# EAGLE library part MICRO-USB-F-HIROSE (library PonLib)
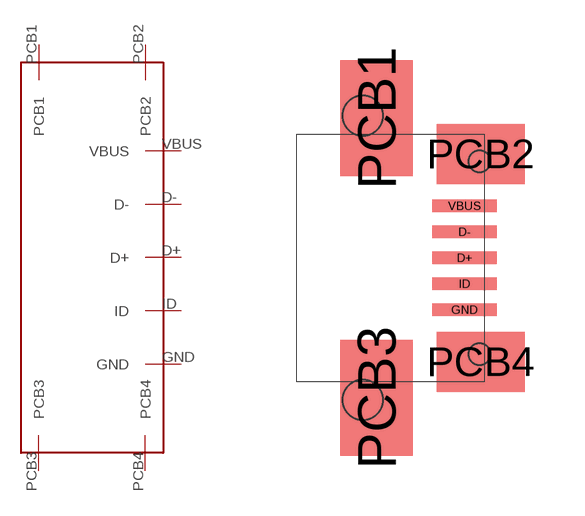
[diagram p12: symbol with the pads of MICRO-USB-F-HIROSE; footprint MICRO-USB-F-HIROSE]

Designator prefix -

## MICRO-USB-F-HIROSE  [MICRO-USB-F-HIROSE]
D+  D+
D-  D-
GND  GND
ID  ID
PCB1  PCB1
PCB2  PCB2
PCB3  PCB3
PCB4  PCB4
VBUS  VBUS

## Footprint MICRO-USB-F-HIROSE (pad centres in mm)
smd 1.6 x 0.305: D+ 2.8,0; D- 2.8,0.65; GND 2.8,-1.3; ID 2.8,-0.65; VBUS 2.8,1.3
smd 1.8 x 2.9: PCB1 0.6,3.5; PCB3 0.6,-3.5
smd 2.2 x 1.5: PCB2 3.2,2.6; PCB4 3.2,-2.6
hole 0.533 at 3.175,2.413
hole 0.533 at 3.175,-2.413
hole 1 at 0.254,-3.556
hole 1 at 0.254,3.556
